(* Logix 5000 AddOnInstructionDefinition export Banner_DFG2_DFG3_PD_v4; software revision 33.00 *)

TYPE Banner_DFG2_DFG3_PDI_v4 :   // UDT that records the converted prcoess data.
STRUCT
   BDC1_Output_State : SINT;   // 0 = Inactive, 1 = Active
   BDC2_Output_State : SINT;   // 0 = Inactive, 1 = Active
   Measurement_Value : INT;
END_STRUCT
END_TYPE

ADD_ON_INSTRUCTION Banner_DFG2_DFG3_PD_v4   (* revision 4.0, vendor Banner Engineering *)
// Takes the raw SINT information and converts that data into actual information.
VAR_INPUT
   SINT0 : SINT; {required}
   SINT1 : SINT; {required}
END_VAR
VAR_IN_OUT
   Process_Data : Banner_DFG2_DFG3_PDI_v4; {required}
END_VAR
VAR_INPUT
   Byte_Swap : BOOL; {required}
END_VAR
VAR
   Temp_Measurement : DINT; {access None}
   Temp_Byte_Array : SINT[2]; {access None}
END_VAR

ROUTINE Logic   (* ladder *)
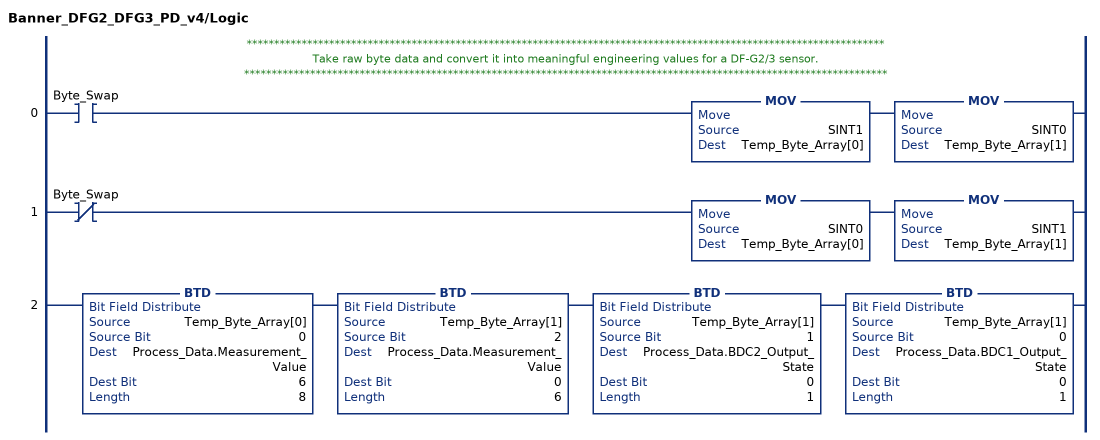
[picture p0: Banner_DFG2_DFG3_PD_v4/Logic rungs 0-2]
   // ********************************************************************************************************************
   // Take raw byte data and convert it into meaningful engineering values for a DF-G2/3 sensor.
   // *********************************************************************************************************************
   0: XIC(Byte_Swap)MOV(SINT1,Temp_Byte_Array[0])MOV(SINT0,Temp_Byte_Array[1]);
   1: XIO(Byte_Swap)MOV(SINT0,Temp_Byte_Array[0])MOV(SINT1,Temp_Byte_Array[1]);
   2: BTD(Temp_Byte_Array[0],0,Process_Data.Measurement_Value,6,8)BTD(Temp_Byte_Array[1],2,Process_Data.Measurement_Value,0,6)BTD(Temp_Byte_Array[1],1,Process_Data.BDC2_Output_State,0,1)BTD(Temp_Byte_Array[1],0,Process_Data.BDC1_Output_State,0,1);
END_ROUTINE
END_ADD_ON_INSTRUCTION
